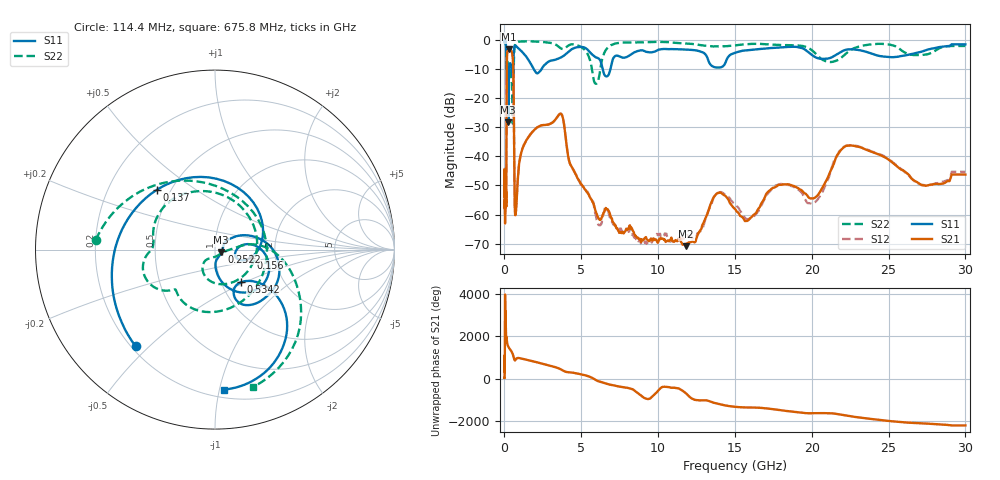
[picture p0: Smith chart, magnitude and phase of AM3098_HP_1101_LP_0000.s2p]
! Date/Time: Thu, Feb 28, 2019 8:45 AM
! Network Analyzer: Agilent Technologies E8364B Rev: A.07.50.67
! Sweep from 0.010 to 30.000 GHz, 1601 Points, Sweep Type: LOG
! Power Supply: 5.022 V, 0.002 A
# Hz S DB R 50
!freq MagS11 AngS11 MagS21 AngS21 MagS12 AngS12 MagS22 AngS22
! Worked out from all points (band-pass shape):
!   1601 points, 10 MHz to 30 GHz, reference 50 ohm
!   highest |S21| = -3.28 dB at 266.5 MHz (marker M1); lowest = -70.9 dB at 11.83 GHz (marker M2)
!   |S21| within 3 dB of the highest: 158.6 MHz to 538.6 MHz (379.9 MHz wide, 109 % of centre)
!   lowest |S11| = -28.4 dB at 250.9 MHz (marker M3), VSWR 1.08, Z = 53.6 - j1.64 ohm
!   |S11| at or under -10 dB: 206.2 MHz to 307.7 MHz (101.5 MHz wide, 39.5 % of centre); 1.889 GHz to 2.425 GHz (535.8 MHz wide, 24.8 % of centre); 6.382 GHz to 6.903 GHz (520.6 MHz wide, 7.84 % of centre)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
!   |S22| runs from -28.8 to -0.5 dB; largest |S21 - S12| = 0.011
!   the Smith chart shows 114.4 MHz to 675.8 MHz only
!   S11 on the Smith chart (normalised r, x): 114.4 MHz: 0.22, -0.45; 137 MHz: 0.42, +0.36; 156 MHz: 1.50, -0.14; 252.2 MHz: 1.08, -0.02; 534.2 MHz: 1.24, -0.48; 675.8 MHz: 0.26, -1.03
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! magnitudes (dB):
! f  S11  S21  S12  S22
! 10 MHz  -0.3  -45.9  -45.9  -0.5
! 38.04 MHz  -0.3  -58.7  -57.5  -0.6
! 114.4 MHz  -3.1  -57.1  -55.6  -3.5
! 137 MHz  -6.7  -24.6  -24.6  -10.5
! 144.7 MHz  -8.7  -14.1  -14.1  -10.0
! 156 MHz  -13.7  -7.0  -7.0  -9.5
! 208.5 MHz  -10.3  -3.9  -3.8  -7.7
! 250.9 MHz  -28.4  -3.3  -3.3  -9.2
! 252.2 MHz  -28.3  -3.3  -3.3  -9.2
! 266.5 MHz  -19.2  -3.3  -3.3  -9.2
! 534.2 MHz  -12.6  -6.0  -6.0  -28.5
! 550.5 MHz  -11.5  -7.2  -7.2  -27.3
! 675.8 MHz  -2.1  -58.6  -57.6  -2.0
! 2.084 GHz  -11.5  -30.3  -30.3  -0.7
! 3.686 GHz  -6.1  -25.5  -25.5  -3.1
! 5.959 GHz  -6.1  -59.2  -60.5  -15.2
! 7.926 GHz  -6.0  -65.0  -64.8  -1.0
! 11.83 GHz  -3.4  -70.9  -67.4  -1.4
! 13.95 GHz  -9.6  -52.6  -52.4  -2.3
! 20.2 GHz  -5.9  -54.2  -55.8  -4.6
! 22.56 GHz  -3.3  -36.3  -36.3  -3.5
! 30 GHz  -1.6  -46.3  -45.3  -2.2
